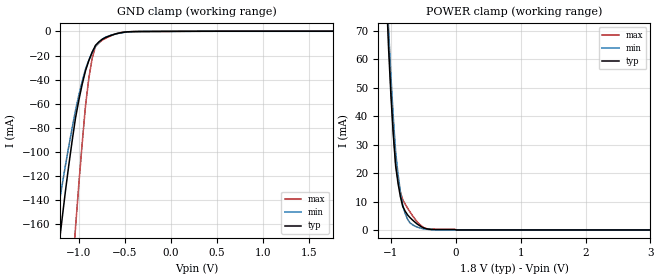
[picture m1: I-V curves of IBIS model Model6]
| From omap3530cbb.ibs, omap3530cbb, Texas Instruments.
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| Model based on original model for BQ0267CS_7LM
|   Sub model BQ0267CS_7LM_PD_ON_1P8
[model]   Model6
|[Input Load]   PD
|[Output Drive]
|Voltage   1.8V
|Mode   INPUT
Model_type   Input
Polarity   Non-Inverting
Vinl =  0.6615
Vinh =  1.2285
C_comp   1.666797p   1.351222p   1.845128p
[Model Spec]
Vinl   0.6615   0.6615   0.6615
Vinh   1.2285   1.2285   1.2285
[Temperature Range]   25   125   -40
[Voltage Range]   1.8   1.62   1.89
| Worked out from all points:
|   GND clamp passes 1 mA (typ) near -0.53 V on its own axis
|   POWER clamp passes 1 mA (typ) near -0.52 V on its own axis
[POWER_clamp]
-1.8V     610.1mA    624.3mA    666.8mA
-1.073V   84.09mA    90.51mA    90.69mA
-1.036V   63.75mA    70.38mA    67.95mA
-1V       47.15mA    53.79mA    49.63mA
-963.6mV  33.38mA    39.44mA    34.81mA
-927.3mV  22.44mA    27.35mA    23.5mA
-890.9mV  16.43mA    19.64mA    17.6mA
-818.2mV  8.271mA    8.652mA    10.62mA
-781.8mV  6.644mA    5.894mA    9.145mA
-636.4mV  2.87mA     1.432mA    4.065mA
-381.8mV  186.8uA    116.6uA    265uA
3.6V      0A         0A         0A
[GND_clamp]
-1.8V     -588mA     -437.3mA   -1.301A
-1.291V   -227.2mA   -178.9mA   -507.7mA
-1.255V   -202.6mA   -161.3mA   -453mA
-1.218V   -178.6mA   -144.2mA   -399.5mA
-1.182V   -155.2mA   -127.4mA   -347.2mA
-1.036V   -71.92mA   -65.58mA   -162.7mA
-927.3mV  -32.62mA   -31.22mA   -61.46mA
-890.9mV  -24.15mA   -23.75mA   -38.57mA
-818.2mV  -11.56mA   -12.34mA   -12.3mA
-709.1mV  -5.034mA   -4.82mA    -5.716mA
-454.5mV  -328.5uA   -434.8uA   -306.2uA
1.764V    137.4uA    69.42uA    248.6uA
